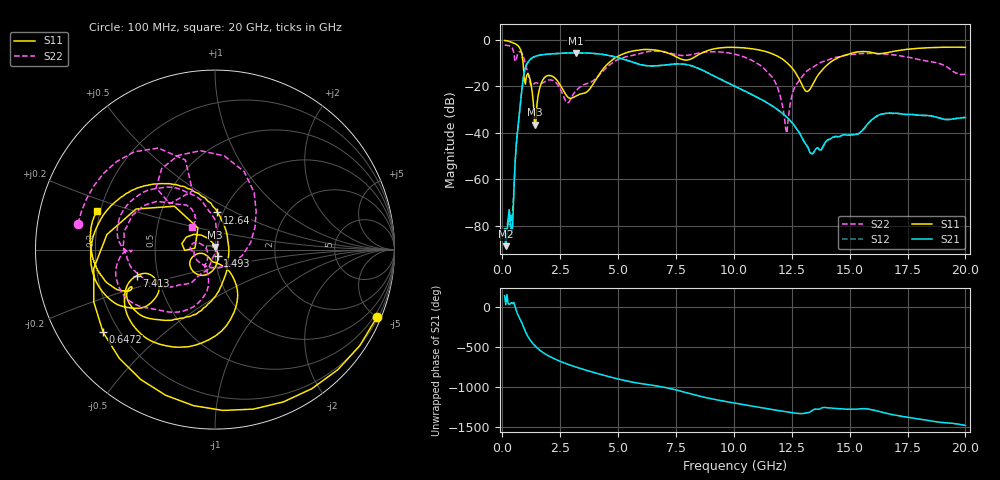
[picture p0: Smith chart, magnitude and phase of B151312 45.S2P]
!  2-Port S-parameters saved by WinCal
! VAR MeasName=S-Parameters (CALIBRATED_DATA) read from VNA (N5244A)
! VAR MeasDate=12/8/2015 5:47:24 PM
! VAR NAME=B151312 45
! VAR FILENAME=B151312 45.S2P
! VAR DATE=12/8/2015 5:47:24 PM
! VAR PHYS_PORTS=1,2
# Hz S DB R 50
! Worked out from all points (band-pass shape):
!   401 points, 100 MHz to 20 GHz, reference 50 ohm
!   highest |S21| = -5.55 dB at 3.184 GHz (marker M1); lowest = -88.9 dB at 149.8 MHz (marker M2)
!   |S21| within 3 dB of the highest: 1.192 GHz to 5.31 GHz (4.119 GHz wide, 127 % of centre)
!   lowest |S11| = -36.5 dB at 1.393 GHz (marker M3), VSWR 1.03, Z = 50.1 + j1.49 ohm
!   |S11| at or under -10 dB: 898.9 MHz to 4.585 GHz (3.686 GHz wide, 134 % of centre); 12.31 GHz to 14.12 GHz (1.802 GHz wide, 13.6 % of centre)
!   |S22| runs from -40.2 to -2.2 dB; largest |S21 - S12| = 0.0017
!   S11 on the Smith chart (normalised r, x): 100 MHz: 0.29, -4.99; 647.2 MHz: 0.14, -0.32; 1.493 GHz: 1.03, -0.07; 7.413 GHz: 0.38, -0.14; 12.64 GHz: 0.94, +0.41; 20 GHz: 0.19, +0.15
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1e8  -0.20 -22.6  -81.38 145.0  -83.03 155.2  -2.19 169.3
1.4975e8  -0.28 -33.5  -88.91 33.9  -81.49 124.3  -2.23 163.9
3.985e8  -0.94 -87.2  -84.04 59.4  -78.15 5.2  -3.02 129.5
6.4725e8  -2.21 -143.5  -40.50 -74.6  -40.51 -74.9  -6.46 133.6
9.955e8  -19.02 175.7  -11.92 59.4  -11.93 59.4  -10.08 42.9
1.3935e9  -36.50 83.9  -7.17 -116.1  -7.18 -116.1  -18.64 -150.2
1.493e9  -28.22 -66.3  -6.83 -144.3  -6.83 -144.3  -18.48 -169.5
1.74175e9  -17.36 -103.1  -6.34 158.8  -6.34 158.7  -18.59 -176.0
2.1895e9  -15.79 -149.9  -5.95 85.2  -5.95 85.1  -17.45 167.7
3.1845e9  -24.17 -111.6  -5.55 -26.3  -5.55 -26.3  -21.89 -123.6
3.43325e9  -23.11 -98.1  -5.58 -49.2  -5.58 -49.2  -19.73 -123.6
4.7765e9  -8.39 -75.2  -7.06 -159.1  -7.05 -159.1  -9.68 -109.3
6.7665e9  -4.58 -148.4  -11.04 93.1  -11.04 93.0  -4.88 -165.8
7.41325e9  -6.73 -161.5  -10.37 54.7  -10.37 54.5  -6.05 -178.9
1.005e10  -3.18 -178.4  -20.01 -117.1  -19.97 -117.3  -6.12 137.9
1.1642e10  -5.89 134.3  -28.29 164.2  -28.32 164.1  -15.88 89.0
1.2239e10  -9.36 109.4  -32.87 135.0  -32.90 135.1  -38.46 17.0
1.2637e10  -13.67 86.3  -37.26 118.5  -37.28 118.5  -20.10 -109.1
1.338325e10  -19.59 -47.7  -49.05 149.7  -48.91 150.6  -11.95 -130.1
1.45275e10  -7.52 -114.8  -41.60 173.1  -41.60 172.9  -7.29 -158.2
1.67165e10  -5.29 -154.9  -31.62 108.1  -31.50 107.6  -6.21 155.1
2e10  -3.19 162.1  -33.41 -35.4  -33.51 -36.0  -14.80 135.5
